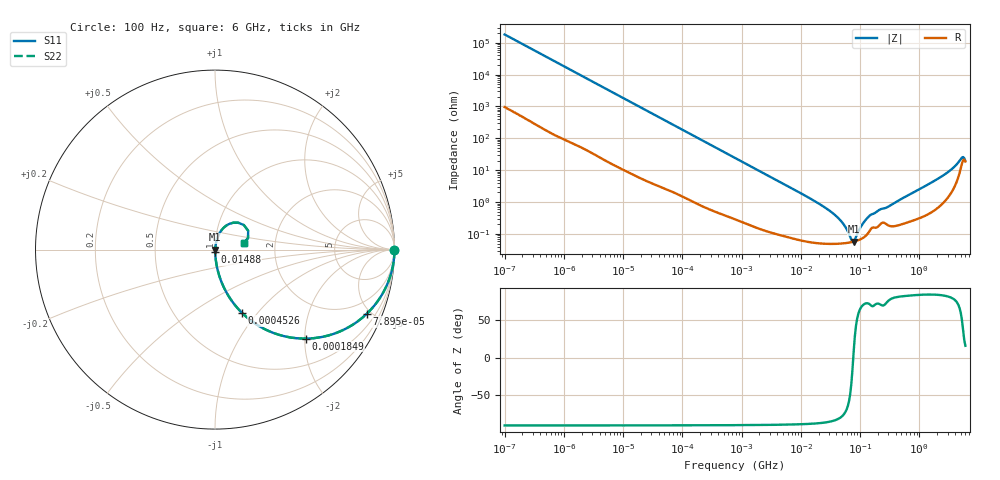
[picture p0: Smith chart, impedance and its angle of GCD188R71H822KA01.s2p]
!Murata Part Number: GCD188R71H822KA01
!These Parameters are Measured in Series Mode Connection
!Data Generated on Mar 13, 2026
!  o--ll--o
!Port1  Port2
!  o------o
!Operation Temp=25[degC], DC Bias Voltage=0[V]
!Freq. Start=100[Hz] Stop=6[GHz] 401[Steps]
# Hz S RI R 50
!Freq.(Hz) S11(Real) S11(Imag) S21(Real) S21(Imag) S12(Real) S12(Imag) S22(Real) S22(Imag)
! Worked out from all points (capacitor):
!   401 points, 100 Hz to 6 GHz, reference 50 ohm
!   read as one part in series: C = 8.73 nF near 109 Hz
!   lowest |Z| = 57.7 mohm at 77.97 MHz (marker M1)
!   series resonance near 76.82 MHz, so ESL is about 490 pH
!   S11 on the Smith chart (normalised r, x): 100 Hz: open; 78.95 kHz: 1.04, -4.72; 184.9 kHz: 1.02, -2.02; 452.6 kHz: 1.01, -0.83; 14.88 MHz: 1.00, -0.02; 6 GHz: 1.37, +0.10
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100  1 -0.000549  3.2e-06 0.000549  3.2e-06 0.000549  1 -0.000549
2008  0.9998 -0.0109  0.00018 0.0109  0.00018 0.0109  0.9998 -0.0109
12041  0.9954 -0.0648  0.00458 0.0648  0.00458 0.0648  0.9954 -0.0648
40335  0.9537 -0.2068  0.0463 0.2068  0.0463 0.2068  0.9537 -0.2068
78952  0.8459 -0.3572  0.1541 0.3572  0.1541 0.3572  0.8459 -0.3572
184852  0.5061 -0.4958  0.4939 0.4958  0.4939 0.4958  0.5061 -0.4958
452617  0.1496 -0.3516  0.8504 0.3516  0.8504 0.3516  0.1496 -0.3516
774597  0.0584 -0.2286  0.9416 0.2286  0.9416 0.2286  0.0584 -0.2286
2481164  0.00706 -0.0759  0.9929 0.0759  0.9929 0.0759  0.00706 -0.0759
1.487547e7  0.000696 -0.0125  0.9993 0.0125  0.9993 0.0125  0.000696 -0.0125
1.555665e7  0.000676 -0.0119  0.9993 0.0119  0.9993 0.0119  0.000676 -0.0119
4.165952e7  0.0005 -0.00328  0.9995 0.00328  0.9995 0.00328  0.0005 -0.00328
5.449875e7  0.000512 -0.00177  0.9995 0.00177  0.9995 0.00177  0.000512 -0.00177
7.129496e7  0.00055 -0.000378  0.9995 0.000378  0.9995 0.000378  0.00055 -0.000378
7.797396e7  0.000571 7.66e-05  0.9994 -7.66e-05  0.9994 -7.66e-05  0.000571 7.66e-05
1.066761e8  0.000712 0.00172  0.9993 -0.00172  0.9993 -0.00172  0.000712 0.00172
1.395531e8  0.00112 0.00331  0.9989 -0.00331  0.9989 -0.00331  0.00112 0.00331
3.124326e8  0.00184 0.00727  0.9982 -0.00727  0.9982 -0.00727  0.00184 0.00727
2.34314e9  0.0118 0.0608  0.9882 -0.0608  0.9882 -0.0608  0.0118 0.0608
3.8344e9  0.0399 0.1126  0.9601 -0.1126  0.9601 -0.1126  0.0399 0.1126
5.016141e9  0.1291 0.15  0.8709 -0.15  0.8709 -0.15  0.1291 0.15
6e9  0.1595 0.037  0.8405 -0.037  0.8405 -0.037  0.1595 0.037
